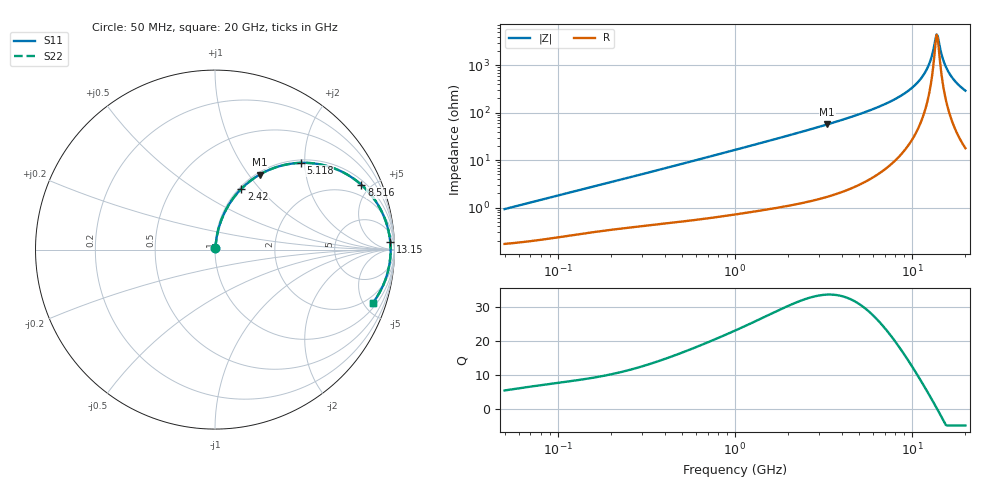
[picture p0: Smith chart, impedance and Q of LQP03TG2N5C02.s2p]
!Murata Part Number: LQP03TG2N5C02
!These Parameters are Measured in Series Mode Connection
!  o--[Z]--o
!Port1  Port2
!  o-------o
!Freq. Start=50[MHz] Stop=20[GHz], 401[Steps]
# Hz S RI R 50
!Freq.(Hz) S11(Real) S11(Imag) S21(Real) S21(Imag) S12(Real) S12(Imag) S22(Real) S22(Imag)
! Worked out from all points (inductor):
!   401 points, 50 MHz to 20 GHz, reference 50 ohm
!   read as one part in series: L = 2.89 nH near 51.52 MHz
!   highest Q = 33.6 at 3.314 GHz (marker M1), where L = 2.72 nH
!   self-resonance near 13.75 GHz
!   S11 on the Smith chart (normalised r, x): 50 MHz: 1.00, +0.02; 2.42 GHz: 1.03, +0.81; 5.118 GHz: 1.06, +1.91; 8.516 GHz: 1.25, +4.40; 13.15 GHz: 19, +36; 20 GHz: 1.36, -5.83
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5e7  0.00179 0.0091  0.9982 -0.0091  0.9982 -0.0091  0.00179 0.0091
1.364002e8  0.00335 0.0238  0.9966 -0.0238  0.9966 -0.0238  0.00335 0.0238
3.721004e8  0.00825 0.0616  0.9918 -0.0616  0.9918 -0.0616  0.00825 0.0616
1e9  0.0329 0.1579  0.9671 -0.1579  0.9671 -0.1579  0.0329 0.1579
2.419936e9  0.1475 0.3393  0.8525 -0.3393  0.8525 -0.3393  0.1475 0.3393
2.728004e9  0.1807 0.3699  0.8193 -0.3699  0.8193 -0.3699  0.1807 0.3699
3.314454e9  0.2493 0.418  0.7507 -0.418  0.7507 -0.418  0.2493 0.418
5.117541e9  0.4769 0.4834  0.5231 -0.4834  0.5231 -0.4834  0.4769 0.4834
7.442007e9  0.7299 0.4219  0.2701 -0.4219  0.2701 -0.4219  0.7299 0.4219
8.516016e9  0.816 0.3606  0.184 -0.3606  0.184 -0.3606  0.816 0.3606
1.004137e10  0.9031 0.2578  0.0969 -0.2578  0.0969 -0.2578  0.9031 0.2578
1.131968e10  0.948 0.1673  0.052 -0.1673  0.052 -0.1673  0.948 0.1673
1.238412e10  0.969 0.0933  0.031 -0.0933  0.031 -0.0933  0.969 0.0933
1.276073e10  0.9734 0.0679  0.0266 -0.0679  0.0266 -0.0679  0.9734 0.0679
1.314879e10  0.9764 0.0423  0.0236 -0.0423  0.0236 -0.0423  0.9764 0.0423
1.354865e10  0.9781 0.0165  0.0219 -0.0165  0.0219 -0.0165  0.9781 0.0165
1.396067e10  0.9784 -0.0094  0.0216 0.0094  0.0216 0.0094  0.9784 -0.0094
1.417136e10  0.978 -0.0223  0.022 0.0223  0.022 0.0223  0.978 -0.0223
1.504638e10  0.9732 -0.0738  0.0268 0.0738  0.0268 0.0738  0.9732 -0.0738
1.597544e10  0.9629 -0.1243  0.0371 0.1243  0.0371 0.1243  0.9629 -0.1243
1.774144e10  0.9326 -0.2086  0.0674 0.2086  0.0674 0.2086  0.9326 -0.2086
2e10  0.8807 -0.2949  0.1193 0.2949  0.1193 0.2949  0.8807 -0.2949
